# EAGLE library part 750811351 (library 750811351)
WE-OLLT Offline Flyback Transformers ETD34 THT; Ui = 85-265V; Uo1 = 36V/3A; f = 100kHz Source: Datasheet
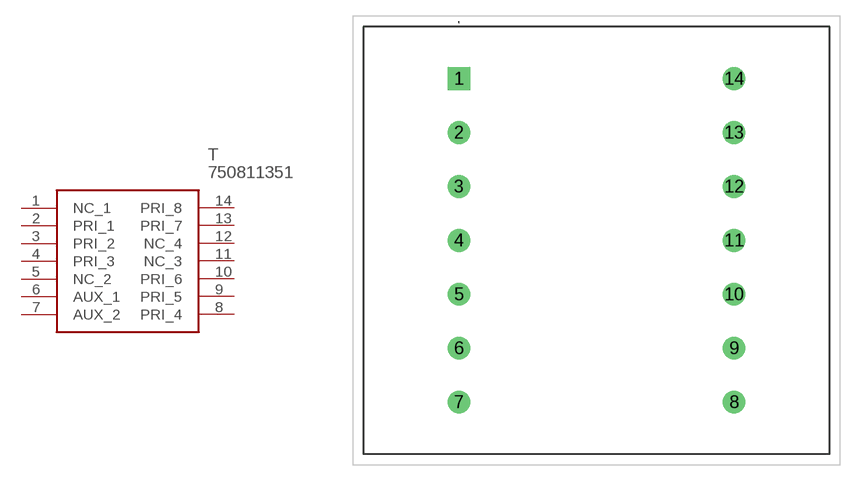
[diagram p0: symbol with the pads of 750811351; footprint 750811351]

Designator prefix T

## 750811351 (Description: WE-OLLT Offline Flyback Transformers ETD34 THT; Ui = 85-265V; Uo1 = 36V/3A; f = 100kHz; Height: 30.48mm; Manufacturer_Name: Wurth Elektronik; Manufacturer_Part_Number: 750811351; Mouser_Part_Number: 710-750811351; Mouser_Price-Stock: https://www.mouser.co.uk/ProductDetail/Wurth-Elektronik/750811351?qs=J4sk5G6CMwbNsr5I5cpBnA%3D%3D)  [750811351]
1  NC_1
2  PRI_1
3  PRI_2
4  PRI_3
5  NC_2
6  AUX_1
7  AUX_2
8  PRI_4
9  PRI_5
10  PRI_6
11  NC_3
12  NC_4
13  PRI_7
14  PRI_8

## Footprint 750811351 (pad centres in mm)
750811351-2
drill 1.4 pad 2.1 square: 1 0,0
drill 1.4 pad 2.1: 2 0,-5; 3 0,-10; 4 0,-15; 5 0,-20; 6 0,-25; 7 0,-30; 8 25.5,-30; 9 25.5,-25; 10 25.5,-20; 11 25.5,-15; 12 25.5,-10; 13 25.5,-5; 14 25.5,0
